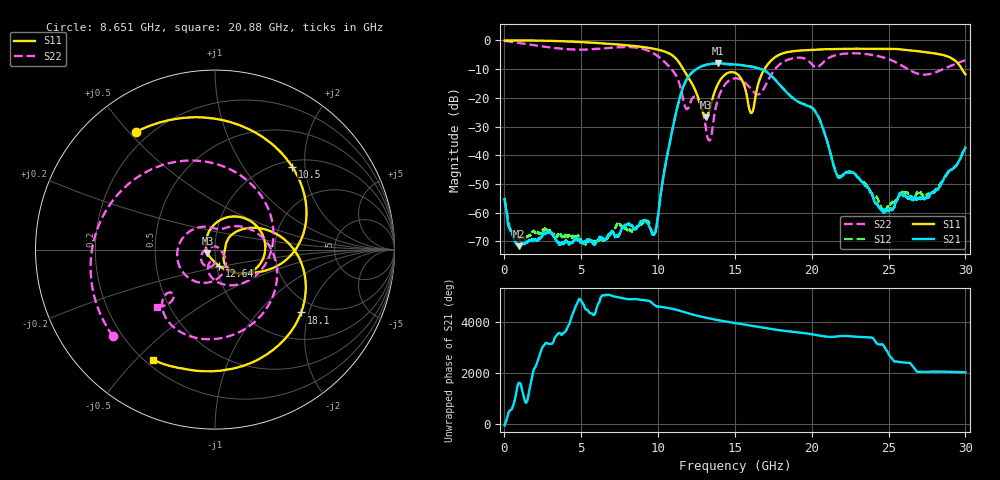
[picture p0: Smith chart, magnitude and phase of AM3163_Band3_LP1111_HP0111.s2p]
!Agilent Technologies,E8364B,MY43040894,A.07.50.67
!Agilent E8364B: A.07.50.67
!Date: Thursday, August 20, 2020 12:16:45
!Correction: S11(Full 2 Port(1,2))
!S21(Full 2 Port(1,2))
!S12(Full 2 Port(1,2))
!S22(Full 2 Port(1,2))
!S2P File: Measurements: S11, S21, S12, S22:
# Hz S  dB  R 50
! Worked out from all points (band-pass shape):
!   3201 points, 10 MHz to 30 GHz, reference 50 ohm
!   highest |S21| = -7.98 dB at 13.9 GHz (marker M1); lowest = -71.7 dB at 937.8 MHz (marker M2)
!   |S21| within 3 dB of the highest: 12.25 GHz to 17.06 GHz (4.814 GHz wide, 32.8 % of centre)
!   lowest |S11| = -26.7 dB at 13.1 GHz (marker M3), VSWR 1.10, Z = 45.9 - j1.75 ohm
!   |S11| at or under -10 dB: 11.63 GHz to 16.92 GHz (5.288 GHz wide, 37 % of centre); 29.78 GHz to end of sweep
!   |S22| runs from -34.9 to -0.2 dB; largest |S21 - S12| = 0.012
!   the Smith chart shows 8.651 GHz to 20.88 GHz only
!   S11 on the Smith chart (normalised r, x): 8.651 GHz: 0.15, +0.52; 10.5 GHz: 1.11, +1.72; 12.64 GHz: 1.03, -0.19; 18.1 GHz: 1.65, -1.78; 20.88 GHz: 0.23, -0.56
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1e7  -0.01 -1.8  -55.27 -64.2  -54.98 -88.9  -0.16 -4.9
9.378156e8  -0.01 -25.3  -71.68 173.6  -69.11 61.1  -0.86 -63.2
2.812191e9  -0.12 -75.9  -66.70 -73.7  -66.29 -63.6  -2.33 -170.9
5.014581e9  -0.57 -133.4  -70.22 152.7  -70.16 168.7  -3.20 73.1
6.682775e9  -1.10 -177.5  -68.45 45.4  -69.05 74.2  -2.67 -20.0
8.650869e9  -2.05 123.8  -64.88 -125.2  -65.02 -125.6  -2.55 -139.6
1.000979e10  -3.22 71.2  -60.68 -62.4  -60.70 -60.1  -5.57 110.3
1.049713e10  -3.99 47.1  -42.74 -93.7  -42.78 -94.7  -7.88 54.0
1.157489e10  -9.47 -18.0  -17.05 112.8  -17.15 113.6  -19.13 -111.1
1.264329e10  -20.50 -75.6  -9.49 -68.2  -9.49 -67.7  -20.85 -149.7
1.310251e10  -26.73 -155.7  -8.52 -131.3  -8.49 -131.2  -30.31 158.5
1.389912e10  -15.15 76.9  -7.98 132.1  -8.09 131.8  -20.39 -50.5
1.5005e10  -11.27 -9.9  -8.38 17.0  -8.46 18.7  -13.20 -145.9
1.608277e10  -25.26 -5.3  -9.15 -87.6  -9.06 -87.1  -17.17 113.2
1.809772e10  -4.52 -36.1  -16.60 78.2  -16.54 78.6  -7.64 -39.4
2.000958e10  -3.31 -98.4  -23.54 -65.3  -23.36 -64.7  -8.34 -137.5
2.088117e10  -3.05 -119.4  -33.11 -153.3  -32.99 -153.1  -6.90 -135.3
2.169652e10  -2.93 -138.5  -47.50 -147.4  -47.17 -144.8  -4.95 -163.8
2.269931e10  -2.87 -160.9  -46.08 -153.4  -46.06 -151.6  -4.47 160.8
2.500479e10  -3.00 144.8  -59.44 -142.5  -57.44 79.5  -6.54 67.7
2.740399e10  -4.08 77.3  -54.92 -105.0  -53.75 -100.9  -11.92 -88.3
3e10  -11.82 -28.6  -37.48 -126.5  -37.01 -129.0  -6.95 130.0
